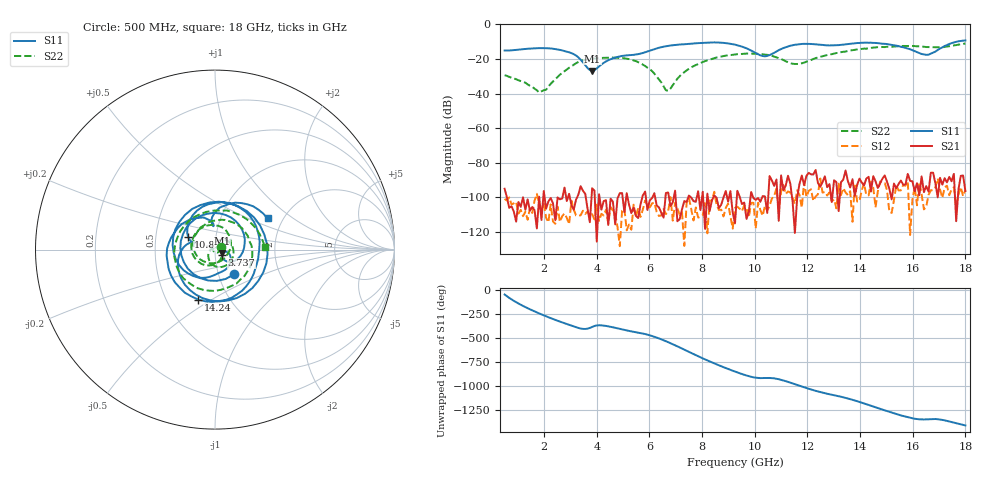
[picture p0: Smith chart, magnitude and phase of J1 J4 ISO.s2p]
!Agilent Technologies,N5230A,MY45001360,A.07.50.67
!Agilent N5230A: A.07.50.67
!Date: Tuesday, April 16, 2024 16:28:17
!Correction: S11(Full 2 Port(1,2))
!S21(Full 2 Port(1,2))
!S12(Full 2 Port(1,2))
!S22(Full 2 Port(1,2))
!S2P File: Measurements: S11, S21, S12, S22:
# Hz S  dB  R 50
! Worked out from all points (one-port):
!   201 points, 500 MHz to 18 GHz, reference 50 ohm
!   lowest |S11| = -26.9 dB at 3.825 GHz (marker M1), VSWR 1.09, Z = 54.1 - j2.28 ohm
!   |S11| at or under -10 dB: start of sweep to 17.69 GHz
!   S11 on the Smith chart (normalised r, x): 500 MHz: 1.19, -0.34; 3.737 GHz: 1.08, -0.06; 10.82 GHz: 0.73, +0.10; 14.24 GHz: 0.72, -0.44; 18 GHz: 1.67, +0.65
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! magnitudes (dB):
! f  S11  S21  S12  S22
! 500 MHz  -15.2  -94.9  -100.8  -29.4
! 1.288 GHz  -14.3  -107.1  -108.2  -33.7
! 1.812 GHz  -13.8  -99.6  -103.9  -39.4
! 2.95 GHz  -16.2  -97.9  -115.4  -25.1
! 3.475 GHz  -22.0  -96.1  -107.7  -20.9
! 3.737 GHz  -26.4  -114.3  -110.4  -20.1
! 3.825 GHz  -26.9  -94.7  -109.6  -19.9
! 4.525 GHz  -20.2  -100.7  -105.5  -19.3
! 5.312 GHz  -17.8  -109.0  -118.6  -20.5
! 6.013 GHz  -15.2  -101.7  -105.7  -25.9
! 6.362 GHz  -13.6  -105.7  -110.7  -31.7
! 6.713 GHz  -12.5  -97.1  -108.0  -38.4
! 7.588 GHz  -11.2  -100.0  -106.7  -24.9
! 9.25 GHz  -11.8  -115.0  -106.0  -17.5
! 10.3 GHz  -18.3  -99.2  -110.6  -17.4
! 10.82 GHz  -15.7  -89.6  -94.9  -19.1
! 11.53 GHz  -11.9  -120.5  -103.6  -23.0
! 12.22 GHz  -11.5  -86.7  -102.0  -20.1
! 14.24 GHz  -10.6  -89.1  -98.7  -14.1
! 15.11 GHz  -11.7  -95.1  -108.4  -13.1
! 16.51 GHz  -17.7  -93.5  -105.4  -13.2
! 18 GHz  -9.4  -96.3  -95.7  -11.1
